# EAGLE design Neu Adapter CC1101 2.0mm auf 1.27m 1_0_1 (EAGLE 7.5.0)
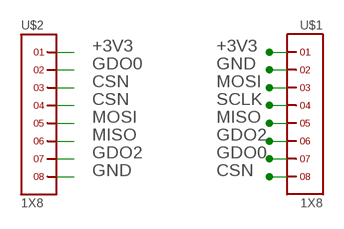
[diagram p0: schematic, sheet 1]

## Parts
U$1  1X8  [1X8]
U$2  1X8  [1X8]

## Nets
+3V3: U$1.1 U$2.1
CSN: U$1.8 U$2.3
GDO0: U$1.7 U$2.2
GDO2: U$1.6 U$2.7
GND: U$1.2 U$2.8
MISO: U$1.5 U$2.6
MOSI: U$1.3 U$2.5
SCLK: U$1.4 U$2.4

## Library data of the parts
U$1 = headers(2mm):1X8
U$2 = headers(.05in):1X8

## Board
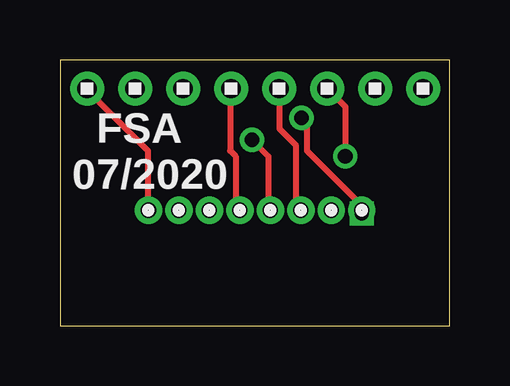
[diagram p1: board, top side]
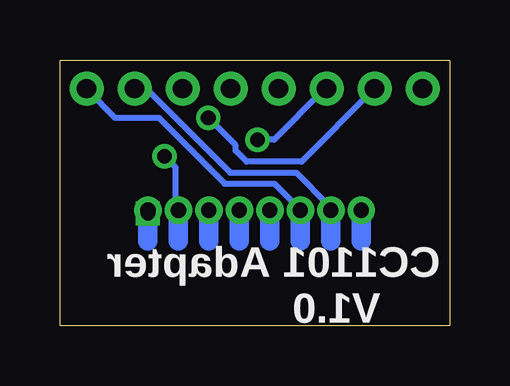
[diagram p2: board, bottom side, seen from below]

Size 16.24 x 11.1 mm. Coordinates in mm from the lower left corner, seen from the top.
Outline: 0,0 16.24,0 16.24,11.1 0,11.1 0,0
Copper layers (1*16): Top 0.035mm / dielectric 1.5mm / Bottom 0.035mm
Design rules "default": minimum track width 10mil, minimum drill 24mil, track to track 8mil, track to pad 8mil, pad to pad 8mil, via to via 8mil, smd to smd 8mil, copper to edge 40mil, drill to drill 8mil, minimum pad ring 10mil, minimum via ring 8mil, stop-mask expansion 4mil, vias tented up to drill 0mil, thermal gap 10mil

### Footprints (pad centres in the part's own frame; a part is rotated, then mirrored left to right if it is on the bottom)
1X8 = drill 0.8 pad 1.422: 1 -7,0; 2 -5,0; 3 -3,0; 4 -1,0; 5 1,0; 6 3,0; 7 5,0; 8 7,0
1X8' = drill 0.635 pad 1.016: 1 0,0; 2 1.27,0; 3 2.54,0; 4 3.81,0; 5 5.08,0; 6 6.35,0; 7 7.62,0; 8 8.89,0

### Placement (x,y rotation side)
U$1  8.13,9.91 0 top
U$2  1X8  [1X8']  3.68,4.83 0 top

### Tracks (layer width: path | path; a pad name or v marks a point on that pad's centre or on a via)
+3V3
  Top 0.254: U$2.1 3.66,5.03 3.66,7.32 1.14,9.83 U$1.1
CSN
  Bottom 0.254: U$2.3 6.4,5.03 7.32,5.94 9.37,5.94 12.12,8.69 13.95,8.69 15.09,9.83 U$1.8
  Bottom 0.813: U$2.3 6.22,3.56
GDO0
  Bottom 0.254: U$2.2 5.03,5.03 6.4,6.4 9.14,6.4 12.57,9.83 13.03,9.83 U$1.7
  Bottom 0.813: U$2.2 4.95,3.56
GDO2  (via drill 0.61)
  Top 0.254: v11.89,7.09 11.89,9.14 11.2,9.83 U$1.6
  Bottom 0.254: v11.89,7.09 11.43,6.63 11.43,5.03 U$2.7
GND  (via drill 0.61)
  Top 0.254: v10.06,8.69 10.29,8.46 10.29,7.32 12.57,5.03 U$2.8
  Bottom 0.254: v10.06,8.69 8.91,7.54 8.91,7.32 8.46,6.86 6.17,6.86 3.2,9.83 U$1.2
MISO
  Top 0.254: U$2.6 9.83,5.03 9.83,7.54 9.14,8.23 9.14,9.83 U$1.5
MOSI  (via drill 0.61)
  Top 0.254: v8,7.77 8.69,7.09 8.69,5.03 U$2.5
  Bottom 0.254: v8,7.77 7.32,7.77 5.26,9.83 U$1.3
  Bottom 0.813: U$2.5 8.76,3.56
N$1
  Bottom 0.813: 3.68,4.7 3.68,3.56
N$2
  Bottom 0.813: 7.49,4.7 7.49,3.56
N$3
  Bottom 0.813: 10.03,4.7 10.03,3.56
N$4
  Bottom 0.813: 11.3,4.7 11.3,3.56
N$5  (via drill 0.6)
  Top 0.813: 12.7,4.7 v12.57,4.7
  Bottom 0.813: v12.57,4.7 12.57,3.56
SCLK
  Top 0.254: U$2.4 7.32,5.03 7.32,7.09 7.09,7.32 7.09,9.83 U$1.4

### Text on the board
tPlace: FSA / 07/2020
bPlace: CC1101 Adapter / V1.0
